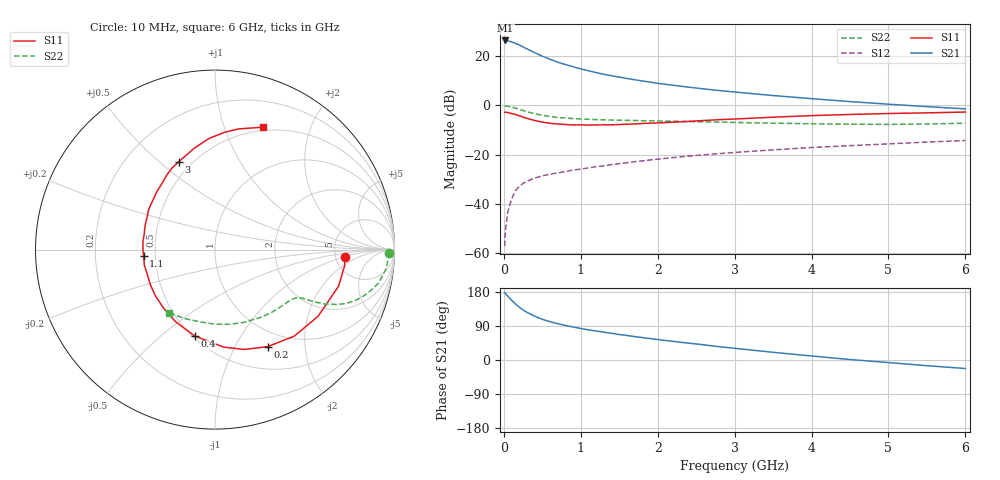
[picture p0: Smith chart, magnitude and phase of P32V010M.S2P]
! SIEMENS Small Signal Semiconductors
! BFP181
! Si NPN RF Bipolar Junction Transistor in SOT143
! VCE = 2 V  IC = 10 mA
! Common Emitter S-Parameters:  March  1996
# GHz  S  MA  R  50
!  f  S11  S21  S12  S22
! GHz  MAG  ANG  MAG  ANG  MAG  ANG  MAG  ANG
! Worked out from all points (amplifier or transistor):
!   36 points, 10 MHz to 6 GHz, reference 50 ohm
!   highest |S21| = 26.3 dB at 20 MHz (marker M1)
!   |S21| within 3 dB of that: start of sweep to 274.2 MHz
!   unconditionally stable (mu >= 1): 948.8 MHz to end of sweep
!   at 250 MHz: K = 0.38, MSG = 27.7 dB, |S12| = -31.6 dB
!   at 1.4 GHz: K = 1.17, MAG = 15.5 dB, |S12| = -24.0 dB
!   at 6 GHz: K = 1.04, MAG = 5.2 dB, |S12| = -14.2 dB
!   S11 on the Smith chart (normalised r, x): 10 MHz: 6.02, -1.08; 200 MHz: 0.78, -1.36; 400 MHz: 0.51, -0.66; 1.1 GHz: 0.43, -0.04; 3 GHz: 0.43, +0.58; 6 GHz: 0.46, +1.36
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0.01  0.7231 -3.4  20.64 177.7  0.0014 80.1  0.9706 -1.0
0.02  0.7279 -7.0  20.72 175.7  0.0028 84.2  0.9675 -2.3
0.05  0.7182 -16.5  20.43 168.6  0.0068 83.2  0.9614 -6.0
0.1  0.6839 -33.0  19.33 157.9  0.0126 74.0  0.9307 -11.5
0.15  0.6539 -47.5  18.16 148.0  0.0185 67.0  0.8841 -16.1
0.2  0.6151 -61.6  16.81 139.5  0.0228 63.2  0.8366 -19.6
0.25  0.5795 -73.7  15.3 131.9  0.0262 59.0  0.7888 -22.4
0.3  0.5458 -84.8  14.02 126.0  0.029 55.8  0.7459 -24.2
0.4  0.4948 -103.1  11.77 115.5  0.0335 51.8  0.6784 -26.5
0.5  0.4581 -118.6  9.932 107.5  0.0373 49.0  0.6307 -27.6
0.6  0.4336 -131.7  8.636 101.1  0.0402 48.3  0.5953 -28.3
0.7  0.4201 -142.3  7.517 95.8  0.043 48.4  0.5714 -28.8
0.9  0.4018 -159.6  6.066 87.2  0.049 48.1  0.5405 -29.9
1.1  0.3997 -174.7  5.039 79.6  0.0542 48.5  0.5214 -31.2
1.5  0.4092 163.2  3.737 67.3  0.0659 48.8  0.5013 -35.1
1.8  0.4304 149.8  3.126 59.1  0.075 48.3  0.4896 -39.0
2.2  0.4568 135.3  2.558 49.1  0.0874 46.6  0.4773 -44.7
3  0.5294 112.5  1.867 30.9  0.1112 42.2  0.4505 -58.1
3.5  0.5763 101.6  1.585 20.3  0.1255 39.0  0.4368 -68.0
4.5  0.6547 85.5  1.194 1.2  0.1528 31.3  0.4152 -90.5
5.5  0.7055 73.7  0.944 -15.0  0.1805 24.2  0.4203 -114.3
6  0.7327 68.6  0.85 -22.5  0.1941 20.1  0.4348 -126.2
